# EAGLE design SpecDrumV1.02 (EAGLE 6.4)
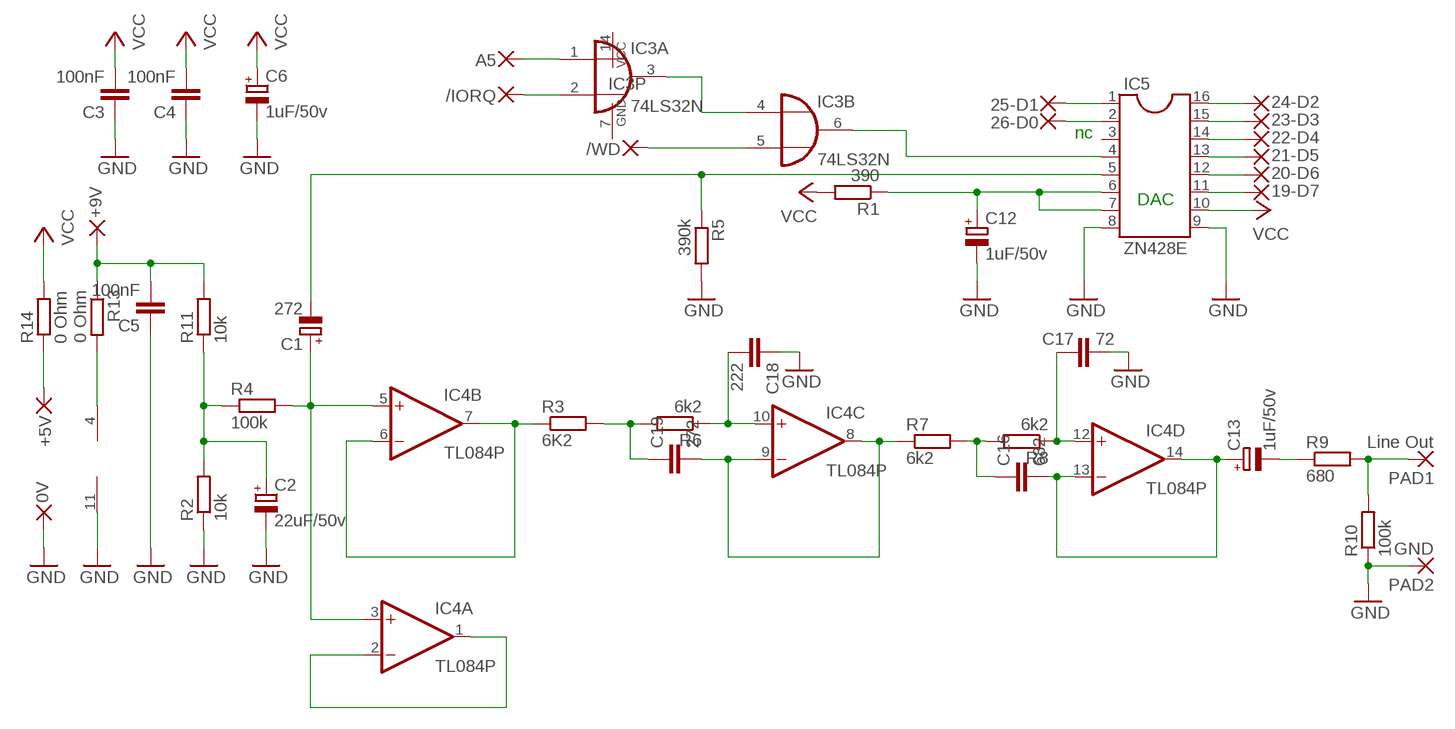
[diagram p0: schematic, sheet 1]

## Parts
0V  1,27-REDONDO0.8  [1,27/0,8-REDONDO]
19-D7  1,27-REDONDO0.8  [1,27/0,8-REDONDO]
20-D6  1,27-REDONDO0.8  [1,27/0,8-REDONDO]
21-D5  1,27-REDONDO0.8  [1,27/0,8-REDONDO]
22-D4  1,27-REDONDO0.8  [1,27/0,8-REDONDO]
23-D3  1,27-REDONDO0.8  [1,27/0,8-REDONDO]
24-D2  1,27-REDONDO0.8  [1,27/0,8-REDONDO]
25-D1  1,27-REDONDO0.8  [1,27/0,8-REDONDO]
26-D0  1,27-REDONDO0.8  [1,27/0,8-REDONDO]
+5V  1,27-REDONDO0.8  [1,27/0,8-REDONDO]
+9V  1,27-REDONDO0.8  [1,27/0,8-REDONDO]
/IORQ  1,27-REDONDO0.8  [1,27/0,8-REDONDO]
/WD  1,27-REDONDO0.8  [1,27/0,8-REDONDO]
A5  1,27-REDONDO0.8  [1,27/0,8-REDONDO]
C1  272  CPOL-EUTT6D6  [TT5D6]
C2  22uF/50v  CPOL-EUE5-5  [E5-5]
C3  100nF  C-EU050-024X044  [C050-024X044]
C4  100nF  C-EU050-024X044  [C050-024X044]
C5  100nF  C-EU050-024X044  [C050-024X044]
C6  1uF/50v  CPOL-EUTT6D6  [TT5D6]
C12  1uF/50v  CPOL-EUTT6D6  [TT5D6]
C13  1uF/50v  CPOL-EUTT6D6  [TT5D6]
C16  682  C-EU050-024X044  [C050-024X044]
C17  72  C-EU050-024X044  [C050-024X044]
C18  222  C-EU050-024X044  [C050-024X044]
C19  272  C-EU050-024X044  [C050-024X044]
IC3  74LS32N  [DIL14]
IC4  TL084P  [DIL14]
IC5  ZN428E  DIL16  [DIL16]
PAD1  Line Out  2,54/1,0  [2,54/1,0]
PAD2  GND  2,54/1,0  [2,54/1,0]
R1  390  R-EU_0207/12  [0207/12]
R2  10k  R-EU_0207/12  [0207/12]
R3  6K2  R-EU_0207/12  [0207/12]
R4  100k  R-EU_0207/12  [0207/12]
R5  390k  R-EU_0207/12  [0207/12]
R6  6k2  R-EU_0207/12  [0207/12]
R7  6k2  R-EU_0207/12  [0207/12]
R8  6k2  R-EU_0207/12  [0207/12]
R9  680  R-EU_0207/12  [0207/12]
R10  100k  R-EU_0207/12  [0207/12]
R11  10k  R-EU_0207/12  [0207/12]
R13  0 Ohm  R-EU_0207/7  [0207/7]
R14  0 Ohm  R-EU_0207/7  [0207/7]

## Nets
GND: 0V.1(P) C2.- C3.1 C4.1 C5.1 C6.- C12.- C17.2 C18.1 IC4.11(P:V-) IC5.8 IC5.9 PAD2.1(P) R2.1 R5.2 R10.1
N$1: C1.+ IC4.3(A:+IN) IC4.5(B:+IN) R4.2
N$3: C2.+ R2.2 R4.1 R11.1
N$4: IC4.1(A:OUT) IC4.2(A:-IN)
N$6: +9V.1(P) C5.2 IC4.4(P:V+) R11.2 R13.1 R13.2
N$15: A5.1(P) IC3.1(A:I0)
N$16: C13.+ C16.2 IC4.13(D:-IN) IC4.14(D:OUT)
N$17: C19.2 IC4.8(C:OUT) IC4.9(C:-IN) R7.1
N$35: /IORQ.1(P) IC3.2(A:I1)
N$36: /WD.1(P) IC3.5(B:I1)
N$37: IC3.3(A:O) IC3.4(B:I0)
N$38: IC3.6(B:O) IC5.4
N$39: 26-D0.1(P) IC5.2
N$40: 25-D1.1(P) IC5.1
N$41: 24-D2.1(P) IC5.16
N$43: 23-D3.1(P) IC5.15
N$47: 22-D4.1(P) IC5.14
N$48: 21-D5.1(P) IC5.13
N$49: 20-D6.1(P) IC5.12
N$54: 19-D7.1(P) IC5.11
N$75: IC4.6(B:-IN) IC4.7(B:OUT) R3.1
N$79: C12.+ IC5.6 IC5.7 R1.1
N$82: C1.- IC5.5 R5.1
N$83: C13.- R9.1
N$85: PAD1.1(P) R9.2 R10.2
N$86: C17.1 IC4.12(D:+IN) R8.1
N$87: C16.1 R7.2 R8.2
N$88: C19.1 R3.2 R6.2
N$90: C18.2 IC4.10(C:+IN) R6.1
VCC: +5V.1(P) C3.2 C4.2 C6.+ IC5.10 R1.2 R14.1 R14.2
Unconnected: IC3.8(C:O) IC3.9(C:I0) IC3.10(C:I1) IC3.11(D:O) IC3.12(D:I0) IC3.13(D:I1) IC5.3

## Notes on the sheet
- nc
- DAC

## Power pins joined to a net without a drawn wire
GND: IC3.7(P:GND)
VCC: IC3.14(P:VCC)

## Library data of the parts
0V 19-D7 20-D6 21-D5 22-D4 23-D3 24-D2 25-D1 26-D0 +5V +9V /IORQ /WD A5 = wirepad2:1,27-REDONDO
C1 C6 C12 C13 = rcl-2:CPOL-EU: POLARIZED CAPACITOR, European symbol
C2 = rcl:CPOL-EU: POLARIZED CAPACITOR, European symbol
C3-C5 C17 C18 = rcl:C-EU: CAPACITOR, European symbol
C16 C19 = rcl-2:C-EU: CAPACITOR, European symbol
IC3 = 74xx-eu:74*32: Quad 2-input OR gate
IC4 = linear:TL084: OP AMP
IC5 = ic-package:DIL16: Dual In Line
PAD1 PAD2 = wirepad:2,54/1,0: THROUGH-HOLE PAD
R1-R11 R13 R14 = rcl:R-EU_: RESISTOR, European symbol

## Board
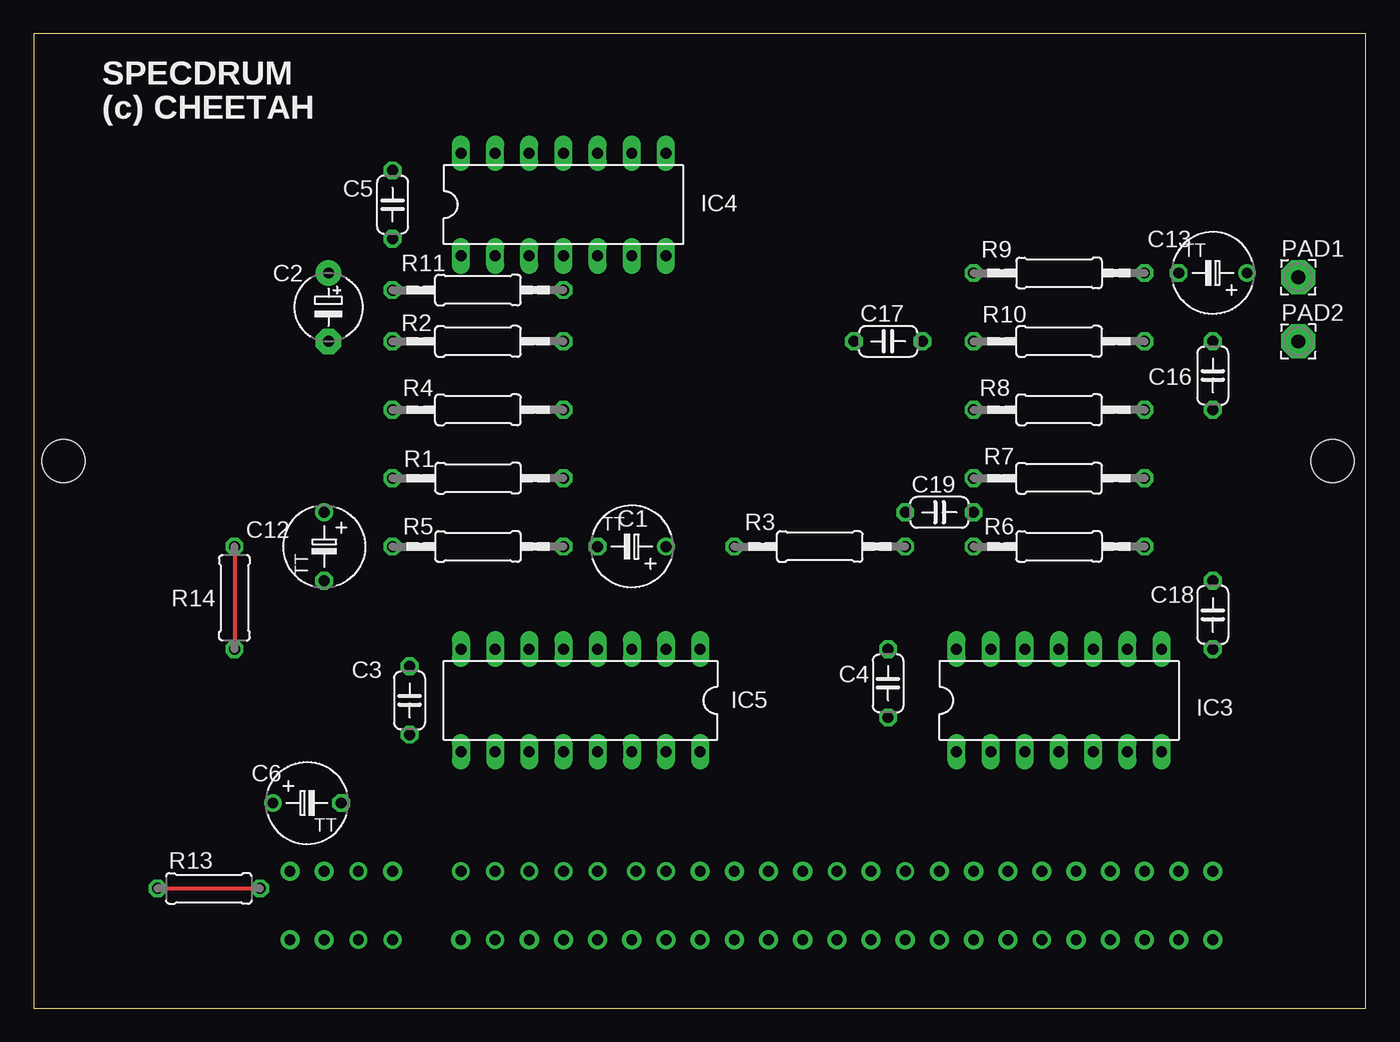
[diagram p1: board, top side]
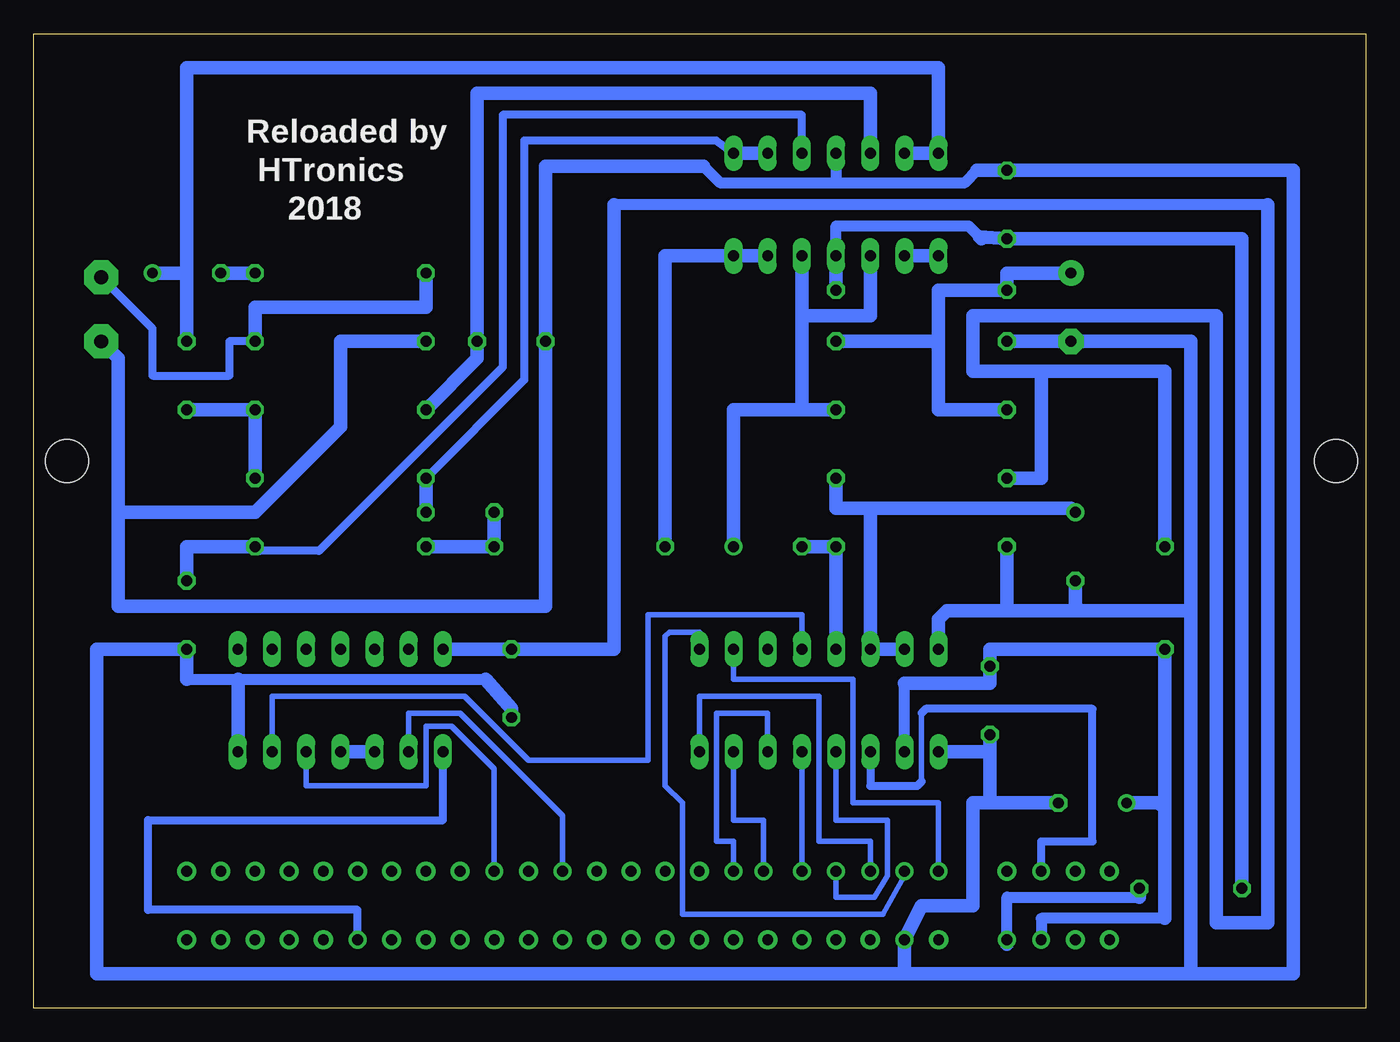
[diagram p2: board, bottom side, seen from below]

Size 99 x 72.39 mm. Coordinates in mm from the lower left corner, seen from the top.
Outline: 0,0 99,0 99,72.39 0,72.39 0,0
Copper layers (1*16): Top 0.035mm / dielectric 1.5mm / Bottom 0.035mm
Design rules "SpecDrum": minimum track width 0.9mm, minimum drill 0.8mm, track to track 0.8mm, track to pad 0.8mm, pad to pad 0.8mm, via to via 0.8mm, smd to smd 8mil, copper to edge 40mil, drill to drill 8mil, minimum pad ring 10mil, minimum via ring 8mil, stop-mask expansion 4mil, vias tented up to drill 0mil, thermal gap 10mil
Holes 3.2 mm at 2.22,40.64 96.52,40.64

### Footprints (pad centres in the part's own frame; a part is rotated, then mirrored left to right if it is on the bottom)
1,27/0,8-REDONDO = drill 0.813 pad 1.27: 1 0,0
TT5D6 = drill 0.813: + -2.54,0 | drill 0.813 octagon: - 2.54,0
E5-5 = drill 0.813 pad 1.905: + -2.54,0 | drill 0.813 pad 1.905 octagon: - 2.54,0
C050-024X044 = drill 0.813 octagon: 1 -2.54,0; 2 2.54,0
DIL14 = drill 0.813 long: 1 -7.62,-3.81; 2 -5.08,-3.81; 3 -2.54,-3.81; 4 0,-3.81; 5 2.54,-3.81; 6 5.08,-3.81; 7 7.62,-3.81; 8 7.62,3.81; 9 5.08,3.81; 10 2.54,3.81; 11 0,3.81; 12 -2.54,3.81; 13 -5.08,3.81; 14 -7.62,3.81
DIL16 = drill 0.813 long: 1 -8.89,-3.81; 2 -6.35,-3.81; 3 -3.81,-3.81; 4 -1.27,-3.81; 5 1.27,-3.81; 6 3.81,-3.81; 7 6.35,-3.81; 8 8.89,-3.81; 9 8.89,3.81; 10 6.35,3.81; 11 3.81,3.81; 12 1.27,3.81; 13 -1.27,3.81; 14 -3.81,3.81; 15 -6.35,3.81; 16 -8.89,3.81
2,54/1,0 = drill 1.016 pad 2.54 octagon: 1 0,0
0207/12 = drill 0.813 octagon: 1 -6.35,0; 2 6.35,0
0207/7 = drill 0.813 octagon: 1 -3.81,0; 2 3.81,0

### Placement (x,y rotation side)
0V  34.29,5.08 0 top
19-D7  24.13,10.16 0 top
20-D6  39.37,10.16 180 top
21-D5  41.91,10.16 0 top
22-D4  46.99,10.16 180 top
23-D3  44.77,10.16 0 top
24-D2  36.83,10.16 180 top
25-D1  34.29,10.16 0 top
26-D0  31.75,10.16 180 top
+5V  24.13,5.08 0 top
+9V  26.67,5.08 0 top
/IORQ  59.69,10.16 0 top
/WD  64.77,10.16 0 top
A5  74.93,5.08 0 top
C1  44.45,34.29 180 top
C2  21.91,52.07 270 top
C3  27.94,22.86 90 top
C4  63.5,24.13 90 top
C5  26.67,59.69 270 top
C6  20.32,15.24 0 top
C12  21.59,34.29 270 top
C13  87.63,54.61 180 top
C16  87.63,46.99 90 top
C17  63.5,49.53 180 top
C18  87.63,29.21 90 top
C19  67.31,36.83 0 top
IC3  76.2,22.86 0 top
IC4  39.37,59.69 0 top
IC5  40.64,22.86 180 top
PAD1  93.98,54.29 0 top
PAD2  93.98,49.53 0 top
R1  33.02,39.37 180 top
R2  33.02,49.53 0 top
R3  58.42,34.29 0 top
R4  33.02,44.45 0 top
R5  33.02,34.29 180 top
R6  76.2,34.29 180 top
R7  76.2,39.37 0 top
R8  76.2,44.45 0 top
R9  76.2,54.61 180 top
R10  76.2,49.53 0 top
R11  33.02,53.34 0 top
R13  13.02,8.89 180 top
R14  14.92,30.48 90 top

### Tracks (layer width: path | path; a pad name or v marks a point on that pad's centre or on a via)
GND
  Bottom 0.813: 28.89,62.23 29.84,61.28 39.37,61.28 | 39.37,61.28 47.94,61.28 49.21,62.55 | 87.63,24.45 83.82,24.45 65.41,24.45 | IC4.11 39.37,61.28
  Bottom 1.016: 34.29,2.54 94.3,2.54 94.3,26.67 C18.1 87.63,24.45 | 34.29,2.54 0V.1 33.02,7.62 29.21,7.62 29.21,15.24 27.94,15.24 | 34.29,2.54 13.02,2.54 | 13.02,2.54 5.4,2.54 5.4,62.23 C5.1 28.89,62.23 | C6.- 27.94,15.24 | C2.- R2.1 13.02,49.53 13.02,29.53 | 13.02,29.53 13.02,2.54 | R5.2 26.67,29.53 | 26.67,29.53 21.27,29.53 | 21.27,29.53 13.02,29.53 | IC5.8 31.75,28.89 31.11,29.53 26.67,29.53 | R10.1 76.2,49.53 76.2,43.18 82.55,36.83 92.71,36.83 | 92.71,36.83 92.71,29.84 60.96,29.84 C17.2 60.96,62.55 49.21,62.55 | 92.71,36.83 92.71,48.26 PAD2.1 | IC5.9 27.94,19.05 | 27.94,19.05 27.94,15.24 | C3.1 27.94,19.05 | C12.- 21.59,29.84 21.27,29.53 | 65.41,24.45 63.5,22.23 C4.1 | IC3.7 83.82,24.45
N$1
  Bottom 1.016: C1.+ 46.99,44.45 41.91,44.45 | 41.91,44.45 R4.2 | IC4.5 41.91,51.44 | 41.91,51.44 41.91,44.45 | IC4.3 36.83,51.44 41.91,51.44
N$2  (via drill 0.8 pad 1.42)
  other vias: 26.67,10.16
N$3
  Bottom 1.016: C2.+ 26.67,54.61 R11.1 31.75,53.34 31.75,49.21 | R4.1 31.75,44.45 31.75,49.21 | R2.2 32.07,49.53 31.75,49.21
N$4
  Bottom 1.016: IC4.1 IC4.2
N$5  (via drill 0.8 pad 1.42)
  other vias: 57.15,10.16
N$6
  Top 0.3: R13.1 R13.2 8.89,8.89
  Bottom 0.813: +9V.1 26.67,8.26 16.83,8.26 | IC4.4 39.37,58.1 29.53,58.1 28.73,57.31
  Bottom 1.016: R13.2 9.21,57.15 C5.2 28.73,57.31 28.57,57.15 | +9V.1 26.67,4.76 | 16.83,8.26 R13.1 | R11.2 IC4.4
N$7  (via drill 0.8 pad 1.42)
  other vias: 21.59,5.08
N$8  (via drill 0.8 pad 1.42)
  other vias: 72.39,5.08
N$15
  Bottom 0.61: A5.1 74.93,7.3 90.49,7.3 90.49,13.97 68.58,13.97 IC3.1
N$16
  Bottom 1.016: C16.2 87.63,54.61 | 87.63,54.61 87.63,69.85 31.75,69.85 IC4.14 IC4.13 | C13.+ 87.63,54.61
N$17
  Bottom 0.61: IC4.8 48.26,64.45 62.55,64.45 62.55,46.67 R7.1
  Bottom 1.016: C19.2 R7.1 | IC4.9 IC4.8
N$21  (via drill 0.8 pad 1.42)
  other vias: 19.05,5.08
N$24  (via drill 0.8 pad 1.42)
  other vias: 21.59,10.16
N$25  (via drill 0.8 pad 1.42)
  other vias: 19.05,10.16
N$26  (via drill 0.8 pad 1.42)
  other vias: 85.09,10.16
N$33  (via drill 0.8 pad 1.42)
  other vias: 82.55,10.16
N$34  (via drill 0.8 pad 1.42)
  other vias: 80.01,10.16
N$35
  Bottom 0.406: IC3.2 71.12,21.91 67.31,21.91 59.69,14.29 /IORQ.1
N$36
  Bottom 0.406: IC3.5 78.74,16.51 69.85,16.51 69.85,20.95 67.94,20.95 64.77,17.78 /WD.1
N$37
  Bottom 1.016: IC3.3 IC3.4
N$38
  Bottom 0.406: IC3.6 81.28,23.18 66.99,23.18 62.23,18.41 53.34,18.41 53.34,29.21 41.91,29.21 IC5.4
N$39
  Bottom 0.406: 26-D0.1 31.75,15.24 38.1,15.24 38.1,24.45 46.99,24.45 IC5.2
N$40
  Bottom 0.406: 25-D1.1 34.29,9.84 35.88,6.99 50.8,6.99 50.8,15.24 52.07,16.51 52.07,27.62 51.75,27.94 49.53,27.94 IC5.1
N$41
  Bottom 0.406: 24-D2.1 36.83,12.38 40.64,12.38 40.64,23.18 49.53,23.18 IC5.16
N$43
  Bottom 0.406: 23-D3.1 44.77,13.97 46.99,13.97 IC5.15
N$47
  Bottom 0.406: 22-D4.1 46.99,12.38 48.26,12.38 48.26,21.91 44.45,21.91 IC5.14
N$48
  Bottom 0.406: 21-D5.1 IC5.13
N$49
  Bottom 0.406: 20-D6.1 39.37,8.26 36.51,8.26 35.56,9.84 35.56,13.97 39.37,13.97 IC5.12
N$54
  Bottom 0.406: 33.02,21.91 33.02,16.83
  Bottom 0.61: IC5.11 36.83,16.51 33.34,16.51 33.02,16.83 | 19-D7.1 24.13,12.38 20.32,12.38 20.32,22.23 32.7,22.23 33.02,21.91
N$63  (via drill 0.8 pad 1.42)
  other vias: 77.47,10.16
N$64  (via drill 0.8 pad 1.42)
  other vias: 74.93,10.16
N$65  (via drill 0.8 pad 1.42)
  other vias: 72.39,10.16
N$66  (via drill 0.8 pad 1.42)
  other vias: 69.85,10.16
N$67  (via drill 0.8 pad 1.42)
  other vias: 67.31,10.16
N$68  (via drill 0.8 pad 1.42)
  other vias: 87.63,10.16
N$69  (via drill 0.8 pad 1.42)
  other vias: 62.23,10.16
N$71  (via drill 0.8 pad 1.42)
  other vias: 54.61,10.16
N$72  (via drill 0.8 pad 1.42)
  other vias: 52.07,10.16
N$73  (via drill 0.8 pad 1.42)
  other vias: 49.53,10.16
N$74  (via drill 0.8 pad 1.42)
  other vias: 31.75,5.08
N$75
  Bottom 1.016: IC4.6 IC4.7 52.07,55.88 R3.1
N$76  (via drill 0.8 pad 1.42)
  other vias: 36.83,5.08
N$77  (via drill 0.8 pad 1.42)
  other vias: 39.37,5.08
N$78  (via drill 0.8 pad 1.42)
  other vias: 41.91,5.08
N$79
  Bottom 1.016: R1.1 39.37,37.15 36.83,37.15 | 36.83,37.15 21.91,37.15 C12.+ | 36.83,37.15 IC5.6 IC5.7
N$80  (via drill 0.8 pad 1.42)
  other vias: 44.45,5.08
N$81  (via drill 0.8 pad 1.42)
  other vias: 46.99,5.08
N$82
  Bottom 1.016: IC5.5 R5.1 C1.-
N$83
  Bottom 1.016: C13.- R9.1
N$84  (via drill 0.8 pad 1.42)
  other vias: 49.53,5.08
N$85
  Bottom 0.61: R10.2 84.45,49.53 84.45,46.99 90.17,46.99 90.17,50.48 PAD1.1
  Bottom 1.016: R9.2 69.85,52.07 82.55,52.07 R10.2
N$86
  Bottom 1.016: IC4.12 36.83,67.94 66.04,67.94 C17.1 66.04,48.26 R8.1
N$87
  Bottom 1.016: R7.2 R8.2 C16.1
N$88
  Bottom 1.016: R6.2 R3.2 C19.1
N$89  (via drill 0.8 pad 1.42)
  other vias: 52.07,5.08
N$90
  Bottom 0.61: IC4.10 41.91,66.36 64.14,66.36 64.14,47.62 77.79,33.97 82.23,33.97 R6.1
  Bottom 1.016: C18.2 87.63,34.29 R6.1
N$91  (via drill 0.8 pad 1.42)
  other vias: 54.61,5.08
N$92  (via drill 0.8 pad 1.42)
  other vias: 57.15,5.08
N$93  (via drill 0.8 pad 1.42)
  other vias: 59.69,5.08
N$94  (via drill 0.8 pad 1.42)
  other vias: 62.23,5.08
N$95  (via drill 0.8 pad 1.42)
  other vias: 64.77,5.08
N$96  (via drill 0.8 pad 1.42)
  other vias: 67.31,5.08
N$97  (via drill 0.8 pad 1.42)
  other vias: 69.85,5.08
N$98  (via drill 0.8 pad 1.42)
  other vias: 87.63,5.08
N$99  (via drill 0.8 pad 1.42)
  other vias: 77.47,5.08
N$100  (via drill 0.8 pad 1.42)
  other vias: 80.01,5.08
N$101  (via drill 0.8 pad 1.42)
  other vias: 82.55,5.08
N$102  (via drill 0.8 pad 1.42)
  other vias: 85.09,5.08
VCC
  Top 0.3: R14.2 R14.1
  Bottom 0.813: 7.3,59.69 55.88,59.69 | IC5.10 34.29,24.13 | 14.92,6.67 24.13,6.67 +5V.1
  Bottom 1.016: R14.2 14.92,47.31 24.45,47.31 | 7.3,59.69 7.3,6.35 11.11,6.35 11.11,51.44 29.21,51.44 29.21,47.31 24.45,47.31 | 55.88,59.69 55.88,26.67 C4.2 IC3.14 | 34.29,24.13 27.94,24.13 C3.2 27.94,26.67 R14.1 14.92,14.92 | 14.92,14.92 14.92,6.67 | C6.+ 15.56,15.24 14.92,14.92 | R1.2 24.13,39.37 24.13,46.99 24.45,47.31

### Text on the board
tNames: SPECDRUM | (c) CHEETAH
bNames: Reloaded by | HTronics | 2018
